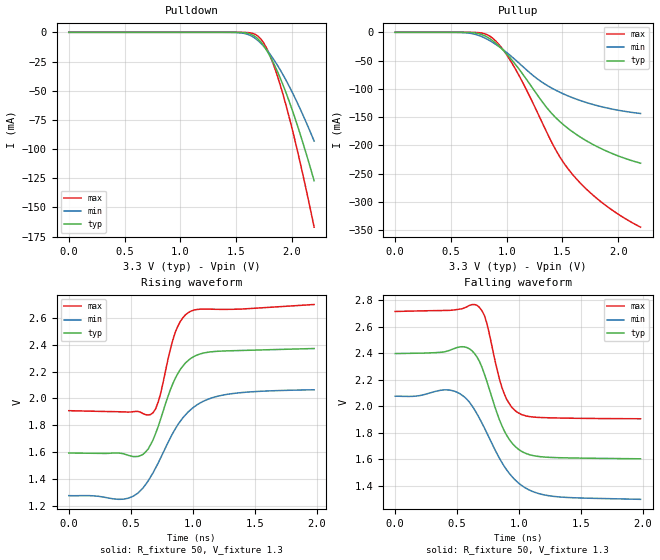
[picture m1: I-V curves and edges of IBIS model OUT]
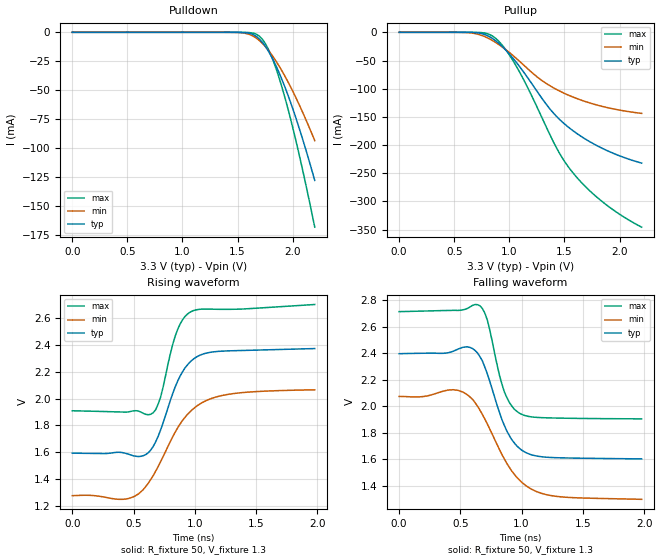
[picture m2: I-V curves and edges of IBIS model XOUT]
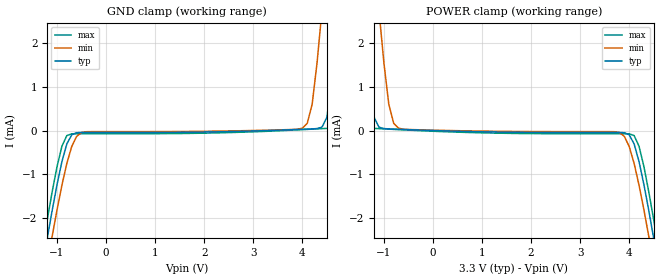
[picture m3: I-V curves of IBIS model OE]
|   IBIS File sg7050ean_33v.ibs
[IBIS Ver]   3.2
[File name]   sg7050ean_33v.ibs
[File Rev]   1.0
[Date]   May 1, 2013
[Source]
[Disclaimer]
Seiko Epson Corporation makes no warranty with respect to the information
contained herein.
[Copyright]
Copyright(C) 2013, Seiko Epson Corporation. All rights reserved.
|   Component SG7050EAN 3.3V
[Component]   sg7050ean_33v
[Manufacturer]   Seiko Epson Corporation
[Package]
R_pkg   0.224   NA   NA
L_pkg   5.50n   NA   NA
C_pkg   1.45p   NA   NA
[Pin] signal_name   model_name   R_pin   L_pin   C_pin
1   OE   OE
2   GND   GND
3   GND   GND
4   OUT   OUT   0.224   5.50n   1.45p
5   XOUT   XOUT   0.224   5.50n   1.45p
6   VCC   POWER
[Diff Pin] inv_pin vdiff   tdelay_typ
4   5   0   0
| Models and submodels in the file (3): OUT (Output_ECL), XOUT (Output_ECL), OE (Input)
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[Model]   OUT
Model_type Output_ECL
Enable Active-High
Polarity Non-Inverting
Vref=1.3
Vmeas=1.97
Rref=50
Cref=0
C_comp   0.121p   0.121p   0.121p
[Temperature Range] 25   105   -40
[Voltage Range]   3.3   2.97   3.63
[Pullup Reference]  3.3   2.97   3.63
[Pulldown Reference]3.3   2.97   3.63
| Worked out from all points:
|   falling waveform, R_fixture 50, V_fixture 1.3: 20-80 % time 191ps typ, 285ps min, 135ps max; typ from 2.4 V to 1.6 V
|   rising waveform, R_fixture 50, V_fixture 1.3: 20-80 % time 195ps typ, 301ps min, 134ps max; typ from 1.59 V to 2.37 V
[Pullup]
0V        806.4pA    1.204nA    885.9pA
650mV     -183.9uA   -1.088mA   -14.42uA
800mV     -5.844mA   -9.686mA   -2.358mA
875mV     -14.92mA   -17.88mA   -10.58mA
975mV     -32.97mA   -31.78mA   -32.77mA
1.075V    -56.01mA   -48.22mA   -63.86mA
1.375V    -137mA     -95.35mA   -183.2mA
1.45V     -152.9mA   -103.4mA   -211.5mA
1.55V     -169.9mA   -112.4mA   -241.3mA
1.675V    -187mA     -121.6mA   -269.6mA
1.825V    -203.5mA   -130.3mA   -296.4mA
2.2V      -231.3mA   -143.5mA   -344.4mA
[Pulldown]
0V        806.4pA    1.204nA    886.1pA
1.5V      -35.86uA   -170.6uA   -2.87uA
1.625V    -1.377mA   -2.54mA    -437.4uA
1.7V      -6.001mA   -7.329mA   -3.538mA
1.75V     -11.83mA   -12.17mA   -9.458mA
1.8V      -19.66mA   -18.15mA   -18.99mA
1.85V     -29.18mA   -25.08mA   -31.52mA
1.9V      -40.12mA   -32.86mA   -46.41mA
1.975V    -58.8mA    -45.94mA   -72.23mA
2.05V     -79.79mA   -60.5mA    -101.4mA
2.125V    -102.7mA   -76.32mA   -133.1mA
2.2V      -127.1mA   -93.13mA   -166.9mA
[Falling Waveform]
R_fixture=50
V_fixture=1.3
V_fixture_min=0.97
V_fixture_max=1.63
0s        2.398V     2.075V     2.715V
460ps     2.429V     2.118V     2.725V
580ps     2.442V     2.05V      2.751V
660ps     2.372V     1.942V     2.762V
740ps     2.186V     1.797V     2.625V
840ps     1.9V       1.609V     2.209V
880ps     1.814V     1.546V     2.094V
1.02ns    1.659V     1.402V     1.937V
1.28ns    1.612V     1.319V     1.912V
1.98ns    1.603V     1.297V     1.905V
[Rising Waveform]
R_fixture=50
V_fixture=1.3
V_fixture_min=0.97
V_fixture_max=1.63
0s        1.592V     1.275V     1.909V
480ps     1.576V     1.256V     1.898V
600ps     1.583V     1.333V     1.887V
680ps     1.691V     1.445V     1.894V
740ps     1.843V     1.554V     2.033V
860ps     2.152V     1.773V     2.496V
920ps     2.241V     1.855V     2.601V
980ps     2.296V     1.913V     2.649V
1.28ns    2.355V     2.031V     2.665V
1.98ns    2.373V     2.065V     2.701V
[Ramp]
R_load=50
dV/dt_r   4.681E-1/1.952E-10   4.741E-1/3.007E-10   4.755E-1/1.340E-10
dV/dt_f   4.769E-1/1.908E-10   4.672E-1/2.847E-10   4.862E-1/1.346E-10
|[End   OUT
[Model]   XOUT
Model_type Output_ECL
Enable Active-High
Polarity Inverting
Vref=1.3
Vmeas=1.97
Rref=50
Cref=0
C_comp   0.121p   0.121p   0.121p
[Temperature Range] 25   105   -40
[Voltage Range]   3.3   2.97   3.63
[Pullup Reference]  3.3   2.97   3.63
[Pulldown Reference]3.3   2.97   3.63
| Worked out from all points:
|   falling waveform, R_fixture 50, V_fixture 1.3: 20-80 % time 189ps typ, 281ps min, 134ps max; typ from 2.4 V to 1.6 V
|   rising waveform, R_fixture 50, V_fixture 1.3: 20-80 % time 198ps typ, 303ps min, 137ps max; typ from 1.59 V to 2.37 V
[Pullup]
0V        806.1pA    1.204nA    885.8pA
650mV     -183.3uA   -1.086mA   -14.36uA
800mV     -5.845mA   -9.693mA   -2.355mA
875mV     -14.95mA   -17.91mA   -10.6mA
975mV     -33.08mA   -31.85mA   -32.91mA
1.075V    -56.25mA   -48.36mA   -64.24mA
1.375V    -137.6mA   -95.58mA   -184.5mA
1.45V     -153.4mA   -103.6mA   -212.9mA
1.55V     -170.5mA   -112.6mA   -242.5mA
1.675V    -187.6mA   -121.9mA   -270.7mA
1.825V    -204mA     -130.5mA   -297.5mA
2.2V      -232mA     -143.8mA   -345.6mA
[Pulldown]
0V        806.2pA    1.204nA    885.9pA
1.5V      -35.4uA    -168.9uA   -2.82uA
1.625V    -1.366mA   -2.525mA   -432.2uA
1.7V      -5.976mA   -7.308mA   -3.513mA
1.75V     -11.8mA    -12.16mA   -9.427mA
1.8V      -19.66mA   -18.14mA   -18.99mA
1.85V     -29.21mA   -25.1mA    -31.58mA
1.9V      -40.21mA   -32.9mA    -46.57mA
1.975V    -58.99mA   -46.03mA   -72.6mA
2.05V     -80.11mA   -60.65mA   -102mA
2.125V    -103.2mA   -76.55mA   -134mA
2.2V      -127.8mA   -93.44mA   -168.1mA
[Falling Waveform]
R_fixture=50
V_fixture=1.3
V_fixture_min=0.97
V_fixture_max=1.63
0s        2.398V     2.075V     2.715V
480ps     2.432V     2.121V     2.724V
580ps     2.444V     2.069V     2.751V
660ps     2.375V     1.97V      2.759V
720ps     2.245V     1.867V     2.652V
860ps     1.854V     1.601V     2.107V
920ps     1.748V     1.511V     2.002V
1ns       1.669V     1.427V     1.94V
1.28ns    1.612V     1.32V      1.911V
1.98ns    1.603V     1.298V     1.905V
[Rising Waveform]
R_fixture=50
V_fixture=1.3
V_fixture_min=0.97
V_fixture_max=1.63
0s        1.592V     1.274V     1.909V
460ps     1.584V     1.253V     1.901V
580ps     1.573V     1.32V      1.889V
660ps     1.641V     1.423V     1.894V
720ps     1.763V     1.526V     2.006V
800ps     1.984V     1.678V     2.332V
860ps     2.129V     1.781V     2.515V
980ps     2.288V     1.917V     2.654V
1.26ns    2.356V     2.029V     2.666V
1.98ns    2.373V     2.065V     2.703V
[Ramp]
R_load=50
dV/dt_r   4.688E-1/1.982E-10   4.745E-1/3.025E-10   4.764E-1/1.372E-10
dV/dt_f   4.767E-1/1.886E-10   4.663E-1/2.814E-10   4.858E-1/1.336E-10
|[End   XOUT
[Model]   OE
Model_type Input
Vinh=2.31
Vinl=0.99
C_comp   1p   1p   1p
[Temperature Range] 25   105   -40
[Voltage Range]   3.3   2.97   3.63
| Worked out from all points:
|   GND clamp passes 1 mA (typ) near -0.96 V on its own axis
|   POWER clamp passes 1 mA (typ) near -1.29 V on its own axis
[GND Clamp]
-3.3V     -17.57mA   -18.04mA   -17.26mA
-1.2V     -2.461mA   -3.05mA    -2.037mA
-900mV    -706.2uA   -1.243mA   -357.4uA
-700mV    -97.47uA   -363.6uA   -75.17uA
4V        28.29uA    52.07uA    20.09uA
4.2V      37.33uA    598uA      31.32uA
4.4V      76.9uA     2.733mA    42.69uA
4.5V      301.4uA    3.927mA    48.43uA
4.7V      2.34mA     6.316mA    64.36uA
4.8V      3.634mA    7.512mA    145.4uA
5.1V      7.519mA    11.1mA     3.362mA
6.6V      27.04mA    29.13mA    24.22mA
[POWER Clamp]
-3.3V     27.04mA    29.13mA    24.22mA
-1.8V     7.519mA    11.1mA     3.362mA
-1.5V     3.634mA    7.512mA    145.4uA
-1.4V     2.34mA     6.316mA    64.36uA
-1.2V     301.4uA    3.927mA    48.43uA
-1.1V     76.9uA     2.733mA    42.69uA
-900mV    37.33uA    598uA      31.32uA
-700mV    28.29uA    52.07uA    20.09uA
4V        -97.47uA   -363.6uA   -75.17uA
4.2V      -706.2uA   -1.243mA   -357.4uA
4.5V      -2.461mA   -3.05mA    -2.036mA
6.6V      -17.57mA   -18.04mA   -17.26mA
